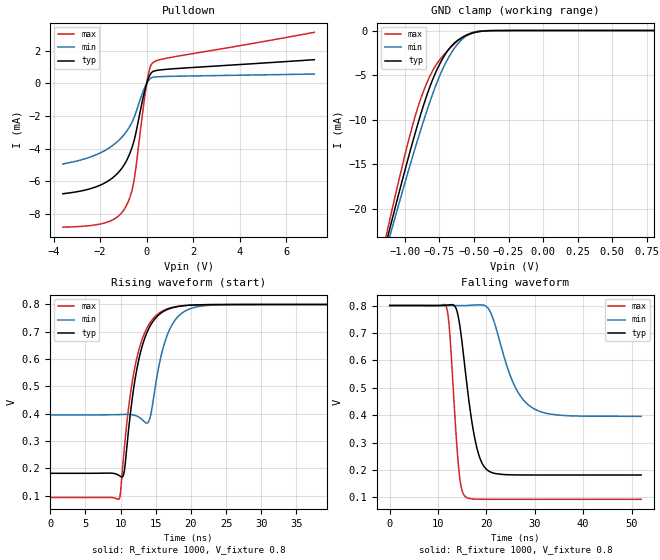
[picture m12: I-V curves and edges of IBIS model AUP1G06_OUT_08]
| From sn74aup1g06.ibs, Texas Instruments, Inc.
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[Model]   AUP1G06_OUT_08
Model_type  Open_drain
Enable   Active-Low
Vref =   0.8
Rref =   1E6
Cref =   30p
Vmeas =   0.4
| variable   typ   min   max
C_comp   1.77pF   1.59pF   1.95pF
| C_pulldown   2.10pF   1.71pF   2.52pF
| C_tri-state   1.77pF   1.59pF   1.95pF
[Temperature Range]   40   100   -40
| Ambient temperature   25   85   -40
[Voltage range]   0.8   0.8   0.8
[Pullup Reference]   0.8   0.8   0.8
[POWER Clamp Reference]   0.8   0.8   0.8
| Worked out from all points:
|   slope of the pulldown table from 0 to 0.12 V, typ, clamps not added: 257 ohm
|   GND clamp passes 1 mA (typ) near -0.61 V on its own axis
|   rising waveform, R_fixture 1000, V_fixture 0.8: 20-80 % time 2.44ns typ, 2.38ns min, 2.49ns max; typ from 0.181 V to 0.8 V
|   falling waveform, R_fixture 1000, V_fixture 0.8: 20-80 % time 2.83ns typ, 4.82ns min, 1.55ns max; typ from 0.8 V to 0.181 V
[GND Clamp]
| AUP1G06_OUT_08
|   Voltage   I(typ)   I(min)   I(max)
-3.6V     -193.5mA   -179.7mA   -210.2mA
-1.13V    -23.52mA   -24.27mA   -22.65mA
-1.11V    -22.29mA   -23.14mA   -21.28mA
-1.09V    -21.07mA   -22.03mA   -19.92mA
-970mV    -13.99mA   -15.5mA    -12.16mA
-870mV    -8.641mA   -10.4mA    -7.007mA
-755mV    -3.984mA   -5.346mA   -3.436mA
-685mV    -2.155mA   -3.063mA   -2.16mA
-625mV    -1.184mA   -1.652mA   -1.265mA
-545mV    -476.4uA   -519uA     -425.6uA
-420mV    -46.16uA   -47.97uA   -21.13uA
800mV     98.86pA    529.8pA    14.12pA
[Pulldown]
| AUP1G06_OUT_08
|   Voltage   I(typ)   I(min)   I(max)
-3.6V     -6.763mA   -4.935mA   -8.814mA
-1.87V    -6.154mA   -4.17mA    -8.58mA
-1.28V    -5.555mA   -3.595mA   -8.209mA
-905mV    -4.84mA    -3.018mA   -7.581mA
-710mV    -4.24mA    -2.594mA   -6.943mA
-570mV    -3.655mA   -2.186mA   -6.156mA
-470mV    -3.08mA    -1.812mA   -5.243mA
-155mV    -882uA     -491.6uA   -1.594mA
15mV      70.31uA    36.95uA    134.1uA
140mV     523.3uA    274.6uA    953.9uA
280mV     740uA      385.5uA    1.291mA
7.2V      1.459mA    578.6uA    3.138mA
[Ramp]
| AUP1G06_OUT_08
| variable   typ   min   max
dV/dt_r   0.38/2.44E-09   0.26/2.40E-09   0.43/2.49E-09
dV/dt_f   0.37/2.84E-09   0.24/4.82E-09   0.43/1.55E-09
R_load = 1000
[Rising Waveform]
| AUP1G06_OUT_08
R_fixture =   1000
C_fixture =   0
L_fixture =   0
V_fixture =   0.8
V_fixture_min = 0.8
V_fixture_max = 0.8
|   Time   V(typ)   V(min)   V(max)
0s        181.5mV    395.5mV    92.72mV
9.8ns     173.3mV    396.7mV    88.2mV
10.51ns   187.8mV    397.2mV    268.6mV
11.35ns   391.1mV    396.9mV    463.4mV
12.31ns   563.3mV    391.1mV    604.3mV
14.06ns   714.9mV    375.3mV    728.5mV
15.99ns   772.9mV    635.4mV    776.7mV
17.94ns   791.6mV    749.2mV    792.6mV
21.07ns   798.7mV    792.5mV    798.8mV
52ns      800mV      800mV      800mV
[Falling Waveform]
| AUP1G06_OUT_08
R_fixture =   1000
C_fixture =   0
L_fixture =   0
V_fixture =   0.8
V_fixture_min = 0.8
V_fixture_max = 0.8
|   Time   V(typ)   V(min)   V(max)
0s        800mV      800mV      800mV
11.69ns   801mV      800mV      796.5mV
12.4ns    802.7mV    800mV      700.6mV
14.32ns   745.7mV    799.8mV    196.3mV
15.71ns   549.2mV    800mV      101.7mV
17.98ns   283.2mV    802.2mV    93.3mV
20.58ns   194.8mV    783.7mV    92.77mV
25.43ns   182mV      522.3mV    92.72mV
29.19ns   181.5mV    430.2mV    92.72mV
52ns      181.5mV    395.5mV    92.72mV
